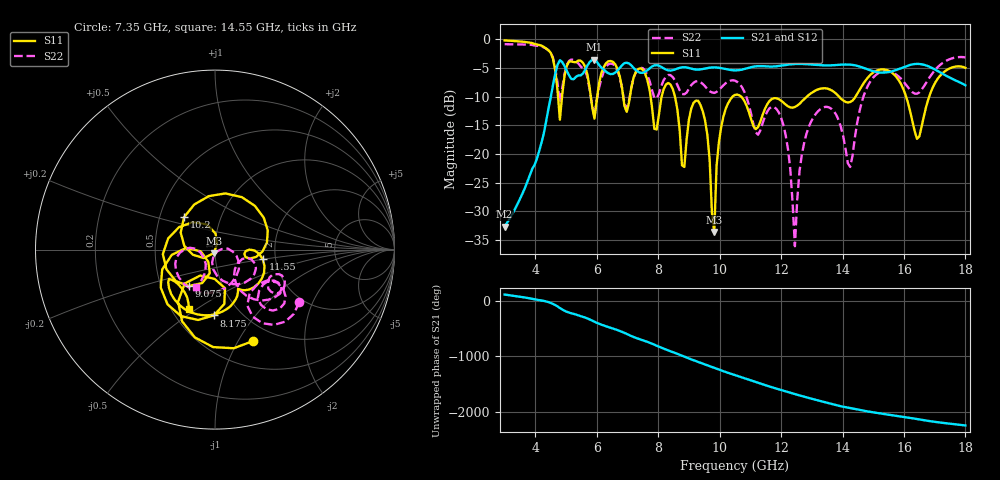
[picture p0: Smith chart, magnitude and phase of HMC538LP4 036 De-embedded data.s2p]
! Chelmsford, MA 01824
! http://www.hittite.com
! Tel: 978-250-3343
! Fax: 978-250-3373
! Device  :  HMC538LP4
! Description:  600 Analog Phase Shifter
! Frequency  :  6.0 GHz - 15.0 GHz
! Package  :  LP4  - 4x4 mm Quad Flatpack No-Lead (QFN) Plastic Package: 24 pin
! Ports  :  2 RF, 1 DC
!  Pin  3  = Rfin  = Port 1
!  Pin  16  = Rfout = Port 2
!  pin  21  = vCTL
! Voltages:  VCTL  = 0 to 5.0 Volts
! Currents :  Vb(V)  Vd(V)  Ib(mA)  Id(mA)
!  0.00  3.60  0.000000	0.476943
! Data:  The device was measured on evaluation board 111296-1.
!  Data was collected using a calibrated network analyzer.
!  The evaluation circuit board was modeled and simulated.This was use
!  to removed the evaluation board circuit from the measured data.
!  The reference plane is the center of the package pin.
! Misc:  Lot #
!Date Measured:  03 - 11 -2009
! Date:  03 - 17 -2009
! Note:
!  Hittite Microwave supplies this data as a sample of measured data at the
!  package pin for this package product.  Your particular data for this product
!  may vary.
!  Data was taken at 25 degrees C.
!  Hittite Microwave reserves the right to change this data at anytime.
# MHz S MA R 50
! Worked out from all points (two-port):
!   201 points, 3 GHz to 18 GHz, reference 50 ohm
!   highest |S21| = -3.52 dB at 5.925 GHz (marker M1); lowest = -32.7 dB at 3 GHz (marker M2)
!   |S21| within 3 dB of the highest: 4.629 GHz to 5.127 GHz (497.5 MHz wide, 10.2 % of centre); 5.324 GHz to 17.44 GHz (12.11 GHz wide, 106 % of centre)
!   lowest |S11| = -33.6 dB at 9.825 GHz (marker M3), VSWR 1.04, Z = 49.3 - j1.94 ohm
!   |S11| at or under -10 dB: 8.547 GHz to 10.42 GHz (1.869 GHz wide, 19.7 % of centre); 10.7 GHz to 12.84 GHz (2.138 GHz wide, 18.2 % of centre); 16.07 GHz to 16.82 GHz (750.7 MHz wide, 4.56 % of centre)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
!   |S22| runs from -36.1 to -0.8 dB; largest |S21 - S12| = 0.0029
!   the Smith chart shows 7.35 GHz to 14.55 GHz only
!   S11 on the Smith chart (normalised r, x): 7.35 GHz: 0.79, -1.16; 8.175 GHz: 0.75, -0.64; 9.075 GHz: 0.69, -0.30; 10.2 GHz: 0.67, +0.26; 11.55 GHz: 1.71, -0.20; 14.55 GHz: 0.61, -0.46
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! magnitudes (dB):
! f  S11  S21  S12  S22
! 3 GHz  -0.2  -32.7  -32.7  -0.8
! 4.8 GHz  -14.0  -3.6  -3.7  -11.0
! 5.55 GHz  -4.1  -6.0  -6.0  -5.1
! 5.925 GHz  -13.8  -3.5  -3.5  -13.5
! 7.35 GHz  -5.2  -5.7  -5.7  -5.1
! 8.025 GHz  -13.1  -4.6  -4.6  -9.5
! 8.175 GHz  -8.7  -5.1  -5.1  -7.1
! 8.775 GHz  -22.0  -4.9  -4.9  -9.5
! 9.075 GHz  -12.1  -5.1  -5.1  -8.0
! 9.525 GHz  -14.1  -5.1  -5.1  -8.2
! 9.825 GHz  -33.6  -4.9  -4.9  -9.3
! 10.2 GHz  -12.1  -5.2  -5.2  -7.6
! 10.5 GHz  -9.7  -5.4  -5.4  -7.2
! 11.55 GHz  -11.3  -4.7  -4.7  -12.6
! 12.15 GHz  -11.4  -4.5  -4.5  -16.7
! 12.45 GHz  -11.8  -4.3  -4.3  -36.1
! 13.05 GHz  -9.1  -4.4  -4.4  -13.6
! 14.25 GHz  -10.9  -4.4  -4.4  -22.3
! 14.55 GHz  -8.9  -4.7  -4.7  -12.6
! 15.53 GHz  -5.5  -5.7  -5.7  -5.6
! 16.43 GHz  -17.3  -4.3  -4.3  -9.5
! 18 GHz  -5.0  -8.0  -8.0  -3.2
